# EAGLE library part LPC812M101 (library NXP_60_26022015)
32-bit ARM Cortex-M0+ microcontroller The LPC81xM are an ARM Cortex-M0+ based, low-cost 32-bit MCU family operating at CPU frequencies of up to 30 MHz. The LPC81xM support up to 16 kB of flash memory and 4 kB of SRAM. The peripheral complement of the LPC81xM includes a CRC engine, one I 2 C-bus interface, up to three USARTs, up to two SPI interfaces, one multi-rate timer, self wake-up timer, and state-configurable timer, one comparator, function-configurable I/O ports through a switch matrix, an input pattern match engine, and up to 18 general-purpose I/O pins. AAL Eindhoven MK
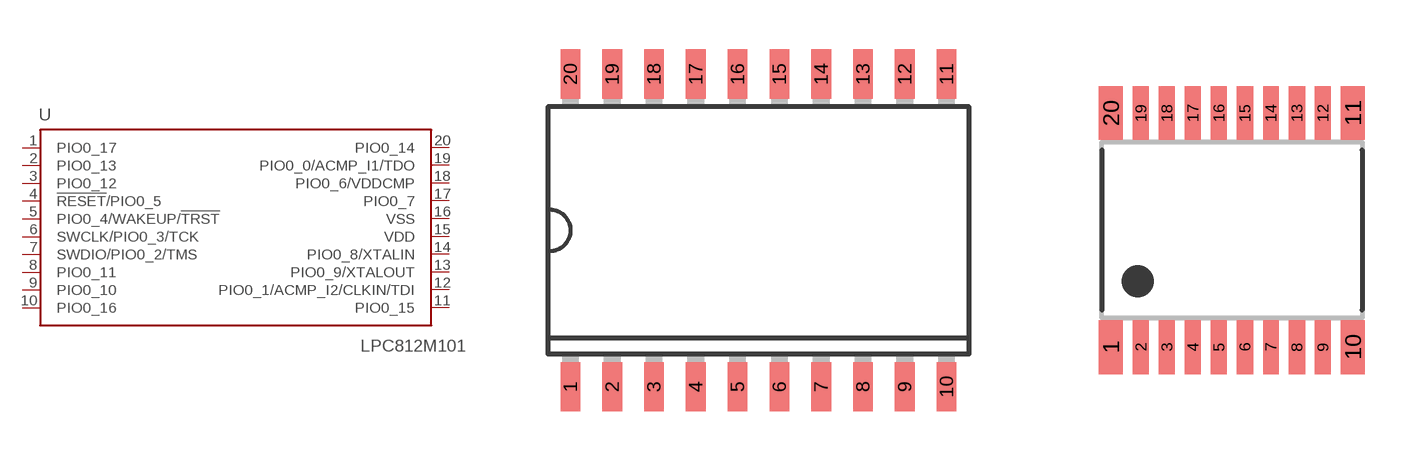
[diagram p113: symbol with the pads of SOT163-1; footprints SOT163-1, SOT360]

Designator prefix U

## LPC812M101JD20 (COMP: 1; FLASH: 16k; GPIO: 18; I2C: 1; SPI: 1; SRAM: 4k; USART: 2)  [SOT163-1]
1  PIO0_17
2  PIO0_13
3  PIO0_12
4  !RESET!/PIO0_5
5  PIO0_4/WAKEUP/!TRST!
6  SWCLK/PIO0_3/TCK
7  SWDIO/PIO0_2/TMS
8  PIO0_11
9  PIO0_10
10  PIO0_16
11  PIO0_15
12  PIO0_1/ACMP_I2/CLKIN/TDI
13  PIO0_9/XTALOUT
14  PIO0_8/XTALIN
15  VDD  pwr
16  VSS  pwr
17  PIO0_7
18  PIO0_6/VDDCMP
19  PIO0_0/ACMP_I1/TDO
20  PIO0_14

## LPC812M101JDH20 (COMP: 1; FLASH: 16k; GPIO: 18; I2C: 1; SPI: 2; SRAM: 4k; USART: 3)  [SOT360]
Pads as for SOT163-1

## Footprint SOT163-1 (pad centres in mm)
SOT163-1 SO20: plastic small outline package; 20 leads; body width 7.5 mm JEDEC: MS-013 IEC: 075E04
smd 0.6 x 1.5: 1 -5.715,-4.75; 2 -4.445,-4.75; 3 -3.175,-4.75; 4 -1.905,-4.75; 5 -0.635,-4.75; 6 0.635,-4.75; 7 1.905,-4.75; 8 3.175,-4.75; 9 4.445,-4.75; 10 5.715,-4.75; 11 5.715,4.75; 12 4.445,4.75; 13 3.175,4.75; 14 1.905,4.75; 15 0.635,4.75; 16 -0.635,4.75; 17 -1.905,4.75; 18 -3.175,4.75; 19 -4.445,4.75; 20 -5.715,4.75

## Footprint SOT360 (pad centres in mm)
SOT360 TSSOP20: plastic thin shrink small outline package; 20 leads; body width 4.4 mm JEDEC: MO-153 IEC:
smd 0.6 x 1.35: 1 -3.025,-2.925; 10 3.025,-2.925; 11 3.025,2.925; 20 -3.025,2.925
smd 0.4 x 1.35: 2 -2.275,-2.925; 3 -1.625,-2.925; 4 -0.975,-2.925; 5 -0.325,-2.925; 6 0.325,-2.925; 7 0.975,-2.925; 8 1.625,-2.925; 9 2.275,-2.925; 12 2.275,2.925; 13 1.625,2.925; 14 0.975,2.925; 15 0.325,2.925; 16 -0.325,2.925; 17 -0.975,2.925; 18 -1.625,2.925; 19 -2.275,2.925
